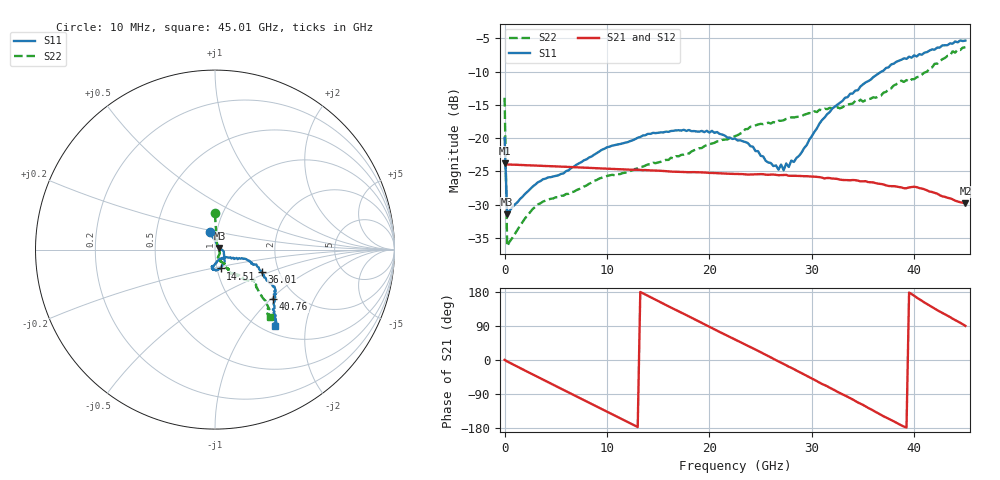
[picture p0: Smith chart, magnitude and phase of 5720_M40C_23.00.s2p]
! Device:  ADRF5720
! Description: 0.5dB LSB GaAs MMIC 6-bit Digital Attenuator
! Frequency:  0.000009 -  40 GHz
! Ports:
!	RF1	= Port 1
!	RF2	= Port 2
! Vdd:  3.3 Volt
! Vss:  -3.3 Volt
! Control:  0/3.3 Volt
! State:  23.00 dB attenuation
! Data:  The device was measured using G-S-G Probes on a matrix board.
!  Data was collected using an calibrated 4 port network analyzer.
!  The reference plane for this measurement is at the launchers.
! Note:  Analog Devices supplies this data as a sample of measured data
!  for this product.  Your particular data for this product may vary.
!  Data was taken at -40 degrees C.
!  Analog Devices reserves the right to change this data at anytime.
# GHZ S DB R 45.0
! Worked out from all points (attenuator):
!   181 points, 10 MHz to 45.01 GHz, reference 45 ohm
!   highest |S21| = -23.78 dB at 10 MHz (marker M1); lowest = -29.8 dB at 45.01 GHz (marker M2)
!   lowest |S11| = -31.4 dB at 260 MHz (marker M3), VSWR 1.05, Z = 47.3 + j0.898 ohm
!   |S11| at or under -10 dB: start of sweep to 36.8 GHz
!   |S22| runs from -36.2 to -6.3 dB; largest |S21 - S12| = 0.00028
!   S11 on the Smith chart (normalised r, x): 10 MHz: 0.93, +0.18; 14.51 GHz: 1.04, -0.22; 36.01 GHz: 1.63, -0.44; 40.76 GHz: 1.53, -1.03; 45.01 GHz: 1.13, -1.36
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0.01  -19.94 106.8  -23.78 0.4  -23.80 0.4  -13.92 90.3
0.26  -31.45 20.8  -23.96 -3.8  -23.98 -3.8  -36.25 32.4
3.26  -26.64 -8.8  -24.14 -45.0  -24.16 -45.0  -29.96 -32.0
7.76  -23.33 -39.4  -24.43 -105.9  -24.45 -106.0  -27.28 -65.7
10.01  -21.37 -51.2  -24.59 -136.4  -24.61 -136.4  -25.69 -70.1
14.51  -19.20 -73.8  -24.86 162.4  -24.88 162.3  -23.70 -69.3
15.26  -19.12 -77.2  -24.91 152.1  -24.93 152.0  -23.56 -67.9
20.26  -18.90 -95.6  -25.23 84.3  -25.25 84.2  -20.81 -58.4
22.76  -20.34 -100.8  -25.39 50.7  -25.42 50.7  -19.56 -58.6
24.01  -21.21 -93.5  -25.47 34.2  -25.49 34.1  -18.28 -57.5
27.01  -23.97 -61.2  -25.56 -6.9  -25.58 -7.0  -17.39 -57.1
27.26  -24.82 -60.2  -25.55 -10.5  -25.57 -10.6  -17.30 -55.5
27.51  -23.81 -53.1  -25.53 -14.2  -25.55 -14.3  -17.10 -56.8
27.76  -24.33 -50.3  -25.66 -17.6  -25.69 -17.7  -16.97 -55.3
28.76  -22.66 -35.6  -25.68 -31.2  -25.70 -31.4  -16.76 -56.6
30.26  -19.07 -24.1  -25.79 -52.2  -25.82 -52.3  -15.96 -56.7
32.01  -15.54 -18.0  -26.08 -76.6  -26.10 -76.7  -15.49 -53.4
36.01  -10.82 -25.2  -26.66 -133.5  -26.69 -133.7  -13.84 -47.0
37.76  -8.91 -31.6  -27.22 -158.3  -27.24 -158.4  -12.51 -45.1
40.76  -7.44 -40.5  -27.58 156.3  -27.62 156.1  -10.44 -40.4
43.76  -5.79 -48.9  -29.20 109.0  -29.22 108.7  -6.94 -47.6
45.01  -5.32 -51.9  -29.82 90.0  -29.85 89.8  -6.34 -50.9
